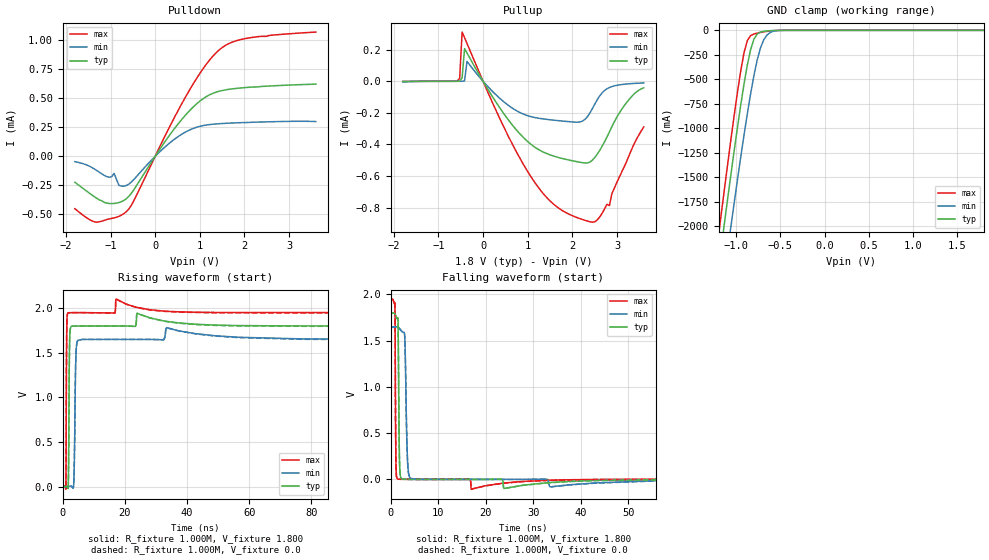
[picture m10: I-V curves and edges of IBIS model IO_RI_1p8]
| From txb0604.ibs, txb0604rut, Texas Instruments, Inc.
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|   Model IO_RI_1p8
[Model] IO_RI_1p8
Model_type 3-state
Polarity   Non-Inverting
Enable   Active-High
Vmeas =  0.900V
Cref =  0.100nF
Rref =  1.000M
Vref =  0.0V
C_comp   3.790pF   3.490pF   3.980pF
[Temperature Range]   27.000   0.125k   -40.000
[Voltage Range]   1.800V   1.650V   1.950V
[Pullup Reference]   1.800V   1.650V   1.950V
[Pulldown Reference]   0.0V   0.0V   0.0V
[POWER Clamp Reference]   1.800V   1.650V   1.950V
[GND Clamp Reference]   0.0V   0.0V   0.0V
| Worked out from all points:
|   slope of the pulldown table from 0 to 0.27 V, typ, clamps not added: 1.76 kohm
|   slope of the pullup table from 0 to 0.27 V, typ, clamps not added: 2.18 kohm
|   GND clamp passes 1 mA (typ) near -0.55 V on its own axis
|   rising waveform, R_fixture 1.000M, V_fixture 1.800: 20-80 % time 229ps typ, 377ps min, 145ps max; typ from 0.003 V to 1.8 V
|   rising waveform, R_fixture 1.000M, V_fixture 0.0: 20-80 % time 229ps typ, 375ps min, 145ps max; typ from 0 V to 1.8 V
|   falling waveform, R_fixture 1.000M, V_fixture 1.800: 20-80 % time 194ps typ, 370ps min, 121ps max; typ from 1.8 V to 0.003 V
|   falling waveform, R_fixture 1.000M, V_fixture 0.0: 20-80 % time 194ps typ, 371ps min, 121ps max; typ from 1.8 V to 0 V
[Pulldown]
|Voltage   I(typ)   I(min)   I(max)
-1.8V     -223.5uA   -46.23uA   -451uA
-1.305V   -362.4uA   -123.2uA   -567.4uA
-1.03V    -406.5uA   -180.3uA   -539.3uA
-920mV    -406uA     -146.5uA   -530.2uA
-810mV    -398uA     -251.2uA   -516.5uA
-590mV    -345.1uA   -239.1uA   -453.6uA
180mV     104.2uA    66.6uA     143.5uA
675mV     353uA      207.9uA    507.5uA
1.115V    507uA      267.5uA    776.9uA
1.5V      566.5uA    282.5uA    936.4uA
2.105V    594.6uA    292.1uA    1.02mA
3.6V      621.5uA    299.5uA    1.07mA
[Pullup]
|Voltage   I(typ)   I(min)   I(max)
-1.8V     -1.708uA   -3.935uA   -871.6nA
-580mV    42.98nA    7.272nA    1.213uA
-525mV    967.3nA    11.84nA    19.05uA
-470mV    21.67uA    150.1nA    311.9uA
-415mV    207.2uA    2.999uA    276.4uA
-360mV    179.1uA    126.1uA    239.6uA
465mV     -205.4uA   -130.1uA   -290.3uA
1.125V    -410.7uA   -227.6uA   -627.5uA
2.17V     -513.2uA   -257.7uA   -870.6uA
2.445V    -500.7uA   -175uA     -893.1uA
2.83V     -320.7uA   -39.6uA    -787.9uA
3.6V      -41.19uA   -10.62uA   -289.3uA
[GND_clamp]
|Voltage   I(typ)   I(min)   I(max)
-1.8V     -6.737A    -7.122A    -6.527A
-1.208V   -2.479A    -2.984A    -2.145A
-1.171V   -2.222A    -2.734A    -1.881A
-1.134V   -1.967A    -2.486A    -1.62A
-1.06V    -1.466A    -1.996A    -1.109A
-912mV    -545.1mA   -1.066A    -226.6mA
-838mV    -197.5mA   -649mA     -54.23mA
-801mV    -91.44mA   -464.4mA   -37.71mA
-727mV    -18.24mA   -180.9mA   -21.59mA
-653mV    -6.339mA   -48.93mA   -10.39mA
-579mV    -1.938mA   -9.115mA   -3.32mA
1.8V      0A         0A         0A
[Ramp]
| variable   typ   min   max
dV/dt_r   1.078/0.223n   0.987/0.371n   1.168/0.145n
dV/dt_f   1.078/0.188n   0.988/0.369n   1.169/0.114n
R_load = 1.000M
[Rising Waveform]
R_fixture= 1.000M
V_fixture= 1.800
V_fixture_min= 1.650
V_fixture_max= 1.950
|time   V(typ)   V(min)   V(max)
0s        3.016mV    4.245mV    2.4mV
980ps     1.89mV     4.267mV    -17.72mV
1.27ns    7.014mV    3.983mV    1.737V
1.67ns    -20.16mV   3.011mV    1.946V
2.23ns    1.656V     6.28mV     1.949V
2.92ns    1.798V     5.251mV    1.949V
3.57ns    1.799V     63.8mV     1.95V
4.18ns    1.799V     1.411V     1.95V
4.84ns    1.8V       1.639V     1.95V
120ns     1.8V       1.65V      1.95V
[Rising Waveform]
R_fixture= 1.000M
V_fixture= 0.0
V_fixture_min= 0.0
V_fixture_max= 0.0
|time   V(typ)   V(min)   V(max)
0s        -2.402uV   10.98uV    -2.986uV
980ps     -1.201mV   39.57uV    -20.31mV
1.27ns    3.827mV    -247.9uV   1.736V
1.67ns    -23.44mV   -1.304mV   1.946V
2.23ns    1.656V     1.787mV    1.949V
2.92ns    1.798V     554.2uV    1.949V
3.57ns    1.799V     58.89mV    1.95V
4.18ns    1.799V     1.409V     1.95V
4.84ns    1.799V     1.639V     1.95V
120ns     1.796V     1.645V     1.947V
[Falling Waveform]
R_fixture= 1.000M
V_fixture= 1.800
V_fixture_min= 1.650
V_fixture_max= 1.950
|time   V(typ)   V(min)   V(max)
0s        1.8V       1.65V      1.95V
880ps     1.791V     1.65V      1.907V
1.11ns    1.766V     1.651V     162.6mV
1.5ns     1.748V     1.647V     2.954mV
1.87ns    173.9mV    1.632V     1.619mV
2.57ns    2.276mV    1.59V      894.4uV
3ns       1.312mV    1.493V     648.3uV
3.58ns    882.3uV    167.7mV    367.8uV
4.18ns    665.7uV    10.51mV    213.9uV
120ns     3.023mV    4.06mV     2.409mV
[Falling Waveform]
R_fixture= 1.000M
V_fixture= 0.0
V_fixture_min= 0.0
V_fixture_max= 0.0
|time   V(typ)   V(min)   V(max)
0s        1.796V     1.645V     1.947V
880ps     1.787V     1.645V     1.904V
1.11ns    1.762V     1.646V     162.1mV
1.5ns     1.744V     1.642V     2.92mV
1.87ns    173.1mV    1.627V     1.588mV
2.57ns    2.23mV     1.585V     865uV
3ns       1.271mV    1.487V     615.5uV
3.58ns    844.5uV    166.3mV    338.8uV
4.18ns    623.4uV    10.38mV    184.9uV
120ns     4.975uV    -161.4uV   5.755uV
